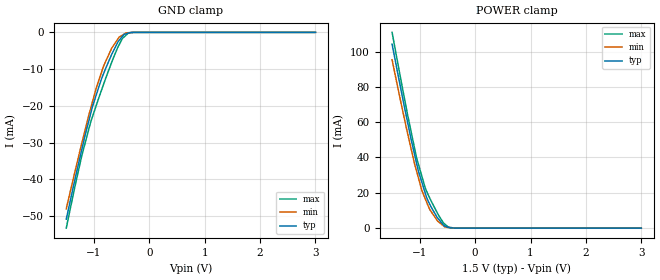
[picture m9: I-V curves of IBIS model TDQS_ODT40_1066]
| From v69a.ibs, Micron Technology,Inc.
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| MODEL TDQS_ODT40_1066 (Termination Model with 40ohm ODT, 800/1066Mbps)
[Model]   TDQS_ODT40_1066
Model_type   Terminator
|   typ   min   max
C_comp   1.25pF   1.10pF   1.45pF
| Note: C_comp changes when the ODT circuit is enabled.
[Voltage Range]   1.5000V   1.4250V   1.5750V
| Junction Temperature (Ambient temp is 35C typ, 95C min, 0C max)
[Temperature Range]   50.0   110.0   0.0
[Add Submodel]
| Submodel Name   Mode
40ohm_ODT_1066   Non-Driving
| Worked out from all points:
|   GND clamp passes 1 mA (typ) near -0.48 V on its own axis
|   POWER clamp passes 1 mA (typ) near -0.53 V on its own axis
[GND Clamp]
|   Voltage   I(typ)   I(min)   I(max)
-1.5V     -50.86mA   -48.03mA   -53.31mA
-1.335V   -39.51mA   -37.41mA   -41.36mA
-1.22V    -31.91mA   -30.23mA   -33.59mA
-1.06V    -22.14mA   -20.74mA   -24.46mA
-1.03V    -20.37mA   -19.08mA   -23.1mA
-960mV    -17.09mA   -15.22mA   -19.96mA
-825mV    -11.18mA   -9.113mA   -14.07mA
-680mV    -6.012mA   -4.321mA   -8.138mA
-565mV    -2.562mA   -1.714mA   -3.942mA
-485mV    -1.053mA   -743.8uA   -1.64mA
-380mV    -208.9uA   -97.58uA   -211uA
3V        0A         0A         0A
[POWER Clamp]
|   Voltage   I(typ)   I(min)   I(max)
-1.5V     104.2mA    95.33mA    110.8mA
-1.22V    59.88mA    53.65mA    64.17mA
-1.06V    36.99mA    32.51mA    40.06mA
-1.025V   32.28mA    28.5mA     36.2mA
-960mV    25.75mA    21.1mA     29.08mA
-875mV    17.23mA    14.62mA    20.76mA
-825mV    13.81mA    10.81mA    17.3mA
-690mV    6.286mA    4.503mA    9.027mA
-565mV    1.438mA    1.112mA    2.719mA
-490mV    520.5uA    387uA      712uA
-290mV    1.769uA    1.056uA    286.1nA
3V        0A         0A         0A
